| IBIS file stm32u575_585_ufbga132.ibs
[IBIS ver] 4.2
[File name] stm32u575_585_ufbga132.ibs
[File Rev] 1.0
[Date]   06-08-2021
[Source] Data Created at STMicroelectronics
[Notes]  File originated from ELDO simulations.
[Disclaimer]  This information is for modeling purpose only and is
   not guaranted. The information is subject to change without
   notice.
[Copyright] Copyright 2021 STMicroelectronics Inc.
|   Component stm32u575_585_ufbga132
[Component] stm32u575_585_ufbga132
[Manufacturer] STMicroelectronics
[Package]
| variable   typ   min   max
R_pkg   0   NA   NA
L_pkg   0   NA   NA
C_pkg   0   NA   NA
[Pin]   signal_name   model_name   R_pin   L_pin   C_pin   | Comment
A1 PE5 io8_100m_hslv_tamp_ft
A10 PC11 io8_100m_hslv_ft
A11 PA15 nc
A12 VDDUSB POWER
A2 PE3 io8_100m_hslv_tamp_ft
A3 PE1 io8_100m_hslv_ft
A4 PB9 io8_100m_i2c_ft
A5 PB6 io8_100m_i2c_ft
A6 PG12 io8_100m_hslv_ft
A7 PD6 io8_166m_hslv_ft
A8 PD5 io8_100m_hslv_ft
A9 PD2 io8_100m_ft
B1 VBAT POWER
B10 PC12 io8_166m_hslv_ft
B11 PC10 io8_100m_ft
B12 PA12 io8_usb_ft
B2 PE4 io8_100m_hslv_tamp_ft
B3 PE2 io8_100m_hslv_ft
B4 PG15 io8_100m_hslv_ft
B5 PH3-BOOT0 io8_100m_ft
B6 PB4 io8_100m_i2c_ft
B7 PG9 io8_100m_hslv_ft
B8 PD4 io8_100m_hslv_ft
B9 PD1 io8_100m_hslv_ft
C1 PC14-OSC32_IN io8_100m_ft
C10 PA13 io8_100m_ft
C11 PA14 io8_100m_ft
C12 PA11 io8_usb_ft
C2 PE6 io8_100m_hslv_tamp_ft
C3 PC13 io8_100m_ft_v33
C4 PE0 io8_100m_hslv_ft
C5 PB8 io8_100m_i2c_ft
C6 PB3 io8_100m_i2c_ft
C7 PG10 io8_100m_hslv_ft
C8 PD3 io8_166m_hslv_ft
C9 PD0 io8_100m_hslv_ft
D1 PC15-OSC32_OUT io8_100m_ft
D10 PA9 io8_100m_usb_vbus_ft
D11 PA10 io8_100m_usb_id
D12 PA8 io8_166m_hslv_ft
D2 PF0 io8_100m_hslv_ft
D3 PF3 io8_100m_hslv_ft
D4 VDD POWER
D5 PB7 io8_166m_hslv_i2c_ft
D6 PB5 io8_166m_hslv_ft
D7 PD7 io8_100m_hslv_ft
D8 VDDIO2 POWER
D9 VDD POWER
E1 PF2 io8_100m_hslv_ft
E10 PC7 io8_100m_ft
E11 PC9 io8_100m_ft
E12 PC8 io8_100m_ft
E2 PF1 io8_100m_hslv_ft
E3 PF4 io8_166m_hslv_ft
E4 VSS GND
E9 VSS GND
F1 PH0-OSC_IN io8_100m_ft
F10 PG7 io8_100m_hslv_ft
F11 PC6 io8_100m_ft
F12 PG8 io8_100m_i2c_ft
F2 PF5 io8_166m_hslv_ft
F3 PC2 io8_100m_hslv_ft
F4 PC3 io8_100m_hslv_ft
F6 VSS GND
F7 VDD POWER
F9 PG6 io8_100m_hslv_ft
G1 PH1-OSC_OUT io8_100m_ft
G10 PG2 io8_100m_hslv_ft
G11 PG3 io8_100m_hslv_ft
G12 PG5 io8_100m_hslv_ft
G2 NRST nc
G3 PC1 io8_166m_hslv_i2c_ft
G4 PA1 io8_100m_hslv_tamp_ft
G6 VDD POWER
G7 VSS GND
G9 PG4 io8_100m_hslv_ft
H1 VSSA GND
H10 PD14 io8_100m_hslv_ft
H11 PD13 io8_100m_hslv_ft
H12 PD15 io8_100m_hslv_ft
H2 PC0 io8_100m_hslv_ft
H3 OPAMP1_VINM nc
H4 VSS GND
H9 VSS GND
J1 VREF+ POWER
J10 PD9 io8_100m_hslv_ft
J11 PD11 io8_100m_hslv_ft
J12 PD12 io8_100m_hslv_ft
J2 PA0 io8_100m_hslv_tamp_ft
J3 PC5 io8_100m_tamp_ft
J4 VDD POWER
J5 PF14 io8_100m_hslv_ft
J6 PE8 io8_100m_hslv_ft
J7 PE10 io8_166m_hslv_ft
J8 PE12 io8_100m_hslv_ft
J9 VDD POWER
K1 VDDA POWER
K10 PB13 io8_100m_i2c_ft
K11 PB14 io8_100m_i2c_ft
K12 PB15 nc
K2 PA2 io8_100m_hslv_ft
K3 PA7 io8_100m_hslv_ft
K4 PB2 io8_100m_hslv_tamp_ft
K5 PF11 io8_166m_hslv_ft
K6 PG1 io8_100m_hslv_ft
K7 PE7 io8_100m_hslv_ft
K8 PE14 io8_100m_hslv_ft
K9 PB10 io8_166m_hslv_i2c_ft
L1 PA3 io8_166m_hslv_ft
L10 VCAP POWER
L11 PB12 io8_166m_hslv_ft
L12 PD8 io8_100m_hslv_ft
L2 PA6 io8_100m_hslv_ft
L3 PA4 io8_100m_hslv_ft
L4 PB1 io8_100m_hslv_ft
L5 PF12 io8_100m_hslv_ft
L6 PF15 io8_100m_hslv_ft
L7 PE11 io8_100m_hslv_ft
L8 PE15 io8_100m_hslv_ft
L9 PB11 io8_100m_hslv_ft
M1 PA5 io8_100m_ft
M10 PG13 io8_100m_hslv_ft
M11 PG11 io8_100m_hslv_ft
M12 PD10 io8_100m_hslv_ft
M2 OPAMP2_VINM nc
M3 PC4 io8_100m_hslv_ft
M4 PB0 io8_100m_hslv_ft
M5 PF13 io8_100m_hslv_ft
M6 PG0 io8_100m_hslv_ft
M7 PE9 io8_166m_hslv_ft
M8 PE13 io8_100m_hslv_ft
M9 PG14 io8_100m_hslv_ft
[Model Selector] io8_100m_ft
io8_100m_ft_hs_1v2  "IO8_FT 100MHz high speed @ 1.2V"
io8_100m_ft_hs_pu_1v2  "IO8_FT 100MHz high speed @ 1.2V pullup"
io8_100m_ft_hs_pd_1v2  "IO8_FT 100MHz high speed @ 1.2V pulldown"
io8_100m_ft_fs_1v2  "IO8_FT 100MHz fast speed @ 1.2V"
io8_100m_ft_fs_pu_1v2  "IO8_FT 100MHz fast speed @ 1.2V pullup"
io8_100m_ft_fs_pd_1v2  "IO8_FT 100MHz fast speed @ 1.2V pulldown"
io8_100m_ft_ms_1v2  "IO8_FT 100MHz med speed @ 1.2V"
io8_100m_ft_ms_pu_1v2  "IO8_FT 100MHz med speed @ 1.2V pullup"
io8_100m_ft_ms_pd_1v2  "IO8_FT 100MHz med speed @ 1.2V pulldown"
io8_100m_ft_ls_1v2  "IO8_FT 100MHz low speed @ 1.2V"
io8_100m_ft_ls_pu_1v2  "IO8_FT 100MHz low speed @ 1.2V pullup"
io8_100m_ft_ls_pd_1v2  "IO8_FT 100MHz low speed @ 1.2V pulldown"
io8_100m_ft_hs_1v8  "IO8_FT 100MHz high speed @ 1.8V"
io8_100m_ft_hs_pu_1v8  "IO8_FT 100MHz high speed @ 1.8V pullup"
io8_100m_ft_hs_pd_1v8  "IO8_FT 100MHz high speed @ 1.8V pulldown"
io8_100m_ft_fs_1v8  "IO8_FT 100MHz fast speed @ 1.8V"
io8_100m_ft_fs_pu_1v8  "IO8_FT 100MHz fast speed @ 1.8V pullup"
io8_100m_ft_fs_pd_1v8  "IO8_FT 100MHz fast speed @ 1.8V pulldown"
io8_100m_ft_ms_1v8  "IO8_FT 100MHz med speed @ 1.8V"
io8_100m_ft_ms_pu_1v8  "IO8_FT 100MHz med speed @ 1.8V pullup"
io8_100m_ft_ms_pd_1v8  "IO8_FT 100MHz med speed @ 1.8V pulldown"
io8_100m_ft_ls_1v8  "IO8_FT 100MHz low speed @ 1.8V"
io8_100m_ft_ls_pu_1v8  "IO8_FT 100MHz low speed @ 1.8V pullup"
io8_100m_ft_ls_pd_1v8  "IO8_FT 100MHz low speed @ 1.8V pulldown"
io8_100m_ft_hs_3v3  "IO8_FT 100MHz high speed @ 3.3V"
io8_100m_ft_hs_pu_3v3  "IO8_FT 100MHz high speed @ 3.3V pullup"
io8_100m_ft_hs_pd_3v3  "IO8_FT 100MHz high speed @ 3.3V pulldown"
io8_100m_ft_fs_3v3  "IO8_FT 100MHz fast speed @ 3.3V"
io8_100m_ft_fs_pu_3v3  "IO8_FT 100MHz fast speed @ 3.3V pullup"
io8_100m_ft_fs_pd_3v3  "IO8_FT 100MHz fast speed @ 3.3V pulldown"
io8_100m_ft_ms_3v3  "IO8_FT 100MHz med speed @ 3.3V"
io8_100m_ft_ms_pu_3v3  "IO8_FT 100MHz med speed @ 3.3V pullup"
io8_100m_ft_ms_pd_3v3  "IO8_FT 100MHz med speed @ 3.3V pulldown"
io8_100m_ft_ls_3v3  "IO8_FT 100MHz low speed @ 3.3V"
io8_100m_ft_ls_pu_3v3  "IO8_FT 100MHz low speed @ 3.3V pullup"
io8_100m_ft_ls_pd_3v3  "IO8_FT 100MHz low speed @ 3.3V pulldown"
[Model Selector] io8_100m_hslv_ft
io8_100m_ft_hs_1v2  "IO8_FT 100MHz high speed @ 1.2V"
io8_100m_ft_hs_pu_1v2  "IO8_FT 100MHz high speed @ 1.2V pullup"
io8_100m_ft_hs_pd_1v2  "IO8_FT 100MHz high speed @ 1.2V pulldown"
io8_100m_ft_fs_1v2  "IO8_FT 100MHz fast speed @ 1.2V"
io8_100m_ft_fs_pu_1v2  "IO8_FT 100MHz fast speed @ 1.2V pullup"
io8_100m_ft_fs_pd_1v2  "IO8_FT 100MHz fast speed @ 1.2V pulldown"
io8_100m_ft_ms_1v2  "IO8_FT 100MHz med speed @ 1.2V"
io8_100m_ft_ms_pu_1v2  "IO8_FT 100MHz med speed @ 1.2V pullup"
io8_100m_ft_ms_pd_1v2  "IO8_FT 100MHz med speed @ 1.2V pulldown"
io8_100m_ft_ls_1v2  "IO8_FT 100MHz low speed @ 1.2V"
io8_100m_ft_ls_pu_1v2  "IO8_FT 100MHz low speed @ 1.2V pullup"
io8_100m_ft_ls_pd_1v2  "IO8_FT 100MHz low speed @ 1.2V pulldown"
io8_100m_ft_hs_1v8  "IO8_FT 100MHz high speed @ 1.8V"
io8_100m_ft_hs_pu_1v8  "IO8_FT 100MHz high speed @ 1.8V pullup"
io8_100m_ft_hs_pd_1v8  "IO8_FT 100MHz high speed @ 1.8V pulldown"
io8_100m_ft_fs_1v8  "IO8_FT 100MHz fast speed @ 1.8V"
io8_100m_ft_fs_pu_1v8  "IO8_FT 100MHz fast speed @ 1.8V pullup"
io8_100m_ft_fs_pd_1v8  "IO8_FT 100MHz fast speed @ 1.8V pulldown"
io8_100m_ft_ms_1v8  "IO8_FT 100MHz med speed @ 1.8V"
io8_100m_ft_ms_pu_1v8  "IO8_FT 100MHz med speed @ 1.8V pullup"
io8_100m_ft_ms_pd_1v8  "IO8_FT 100MHz med speed @ 1.8V pulldown"
io8_100m_ft_ls_1v8  "IO8_FT 100MHz low speed @ 1.8V"
io8_100m_ft_ls_pu_1v8  "IO8_FT 100MHz low speed @ 1.8V pullup"
io8_100m_ft_ls_pd_1v8  "IO8_FT 100MHz low speed @ 1.8V pulldown"
io8_100m_ft_hs_3v3  "IO8_FT 100MHz high speed @ 3.3V"
io8_100m_ft_hs_pu_3v3  "IO8_FT 100MHz high speed @ 3.3V pullup"
io8_100m_ft_hs_pd_3v3  "IO8_FT 100MHz high speed @ 3.3V pulldown"
io8_100m_ft_fs_3v3  "IO8_FT 100MHz fast speed @ 3.3V"
io8_100m_ft_fs_pu_3v3  "IO8_FT 100MHz fast speed @ 3.3V pullup"
io8_100m_ft_fs_pd_3v3  "IO8_FT 100MHz fast speed @ 3.3V pulldown"
io8_100m_ft_ms_3v3  "IO8_FT 100MHz med speed @ 3.3V"
io8_100m_ft_ms_pu_3v3  "IO8_FT 100MHz med speed @ 3.3V pullup"
io8_100m_ft_ms_pd_3v3  "IO8_FT 100MHz med speed @ 3.3V pulldown"
io8_100m_ft_ls_3v3  "IO8_FT 100MHz low speed @ 3.3V"
io8_100m_ft_ls_pu_3v3  "IO8_FT 100MHz low speed @ 3.3V pullup"
io8_100m_ft_ls_pd_3v3  "IO8_FT 100MHz low speed @ 3.3V pulldown"
io8_100m_hslv_ft_hs_1v2  "IO8_FT 100MHz HSLV high speed @ 1.2V"
io8_100m_hslv_ft_hs_pu_1v2  "IO8_FT 100MHz HSLV high speed @ 1.2V pullup"
io8_100m_hslv_ft_hs_pd_1v2  "IO8_FT 100MHz HSLV high speed @ 1.2V pulldown"
io8_100m_hslv_ft_fs_1v2  "IO8_FT 100MHz HSLV fast speed @ 1.2V"
io8_100m_hslv_ft_fs_pu_1v2  "IO8_FT 100MHz HSLV fast speed @ 1.2V pullup"
io8_100m_hslv_ft_fs_pd_1v2  "IO8_FT 100MHz HSLV fast speed @ 1.2V pulldown"
io8_100m_hslv_ft_ms_1v2  "IO8_FT 100MHz HSLV med speed @ 1.2V"
io8_100m_hslv_ft_ms_pu_1v2  "IO8_FT 100MHz HSLV med speed @ 1.2V pullup"
io8_100m_hslv_ft_ms_pd_1v2  "IO8_FT 100MHz HSLV med speed @ 1.2V pulldown"
io8_100m_hslv_ft_ls_1v2  "IO8_FT 100MHz HSLV low speed @ 1.2V"
io8_100m_hslv_ft_ls_pu_1v2  "IO8_FT 100MHz HSLV low speed @ 1.2V pullup"
io8_100m_hslv_ft_ls_pd_1v2  "IO8_FT 100MHz HSLV low speed @ 1.2V pulldown"
io8_100m_hslv_ft_hs_1v8  "IO8_FT 100MHz HSLV high speed @ 1.8V"
io8_100m_hslv_ft_hs_pu_1v8  "IO8_FT 100MHz HSLV high speed @ 1.8V pullup"
io8_100m_hslv_ft_hs_pd_1v8  "IO8_FT 100MHz HSLV high speed @ 1.8V pulldown"
io8_100m_hslv_ft_fs_1v8  "IO8_FT 100MHz HSLV fast speed @ 1.8V"
io8_100m_hslv_ft_fs_pu_1v8  "IO8_FT 100MHz HSLV fast speed @ 1.8V pullup"
io8_100m_hslv_ft_fs_pd_1v8  "IO8_FT 100MHz HSLV fast speed @ 1.8V pulldown"
io8_100m_hslv_ft_ms_1v8  "IO8_FT 100MHz HSLV med speed @ 1.8V"
io8_100m_hslv_ft_ms_pu_1v8  "IO8_FT 100MHz HSLV med speed @ 1.8V pullup"
io8_100m_hslv_ft_ms_pd_1v8  "IO8_FT 100MHz HSLV med speed @ 1.8V pulldown"
io8_100m_hslv_ft_ls_1v8  "IO8_FT 100MHz HSLV low speed @ 1.8V"
io8_100m_hslv_ft_ls_pu_1v8  "IO8_FT 100MHz HSLV low speed @ 1.8V pullup"
io8_100m_hslv_ft_ls_pd_1v8  "IO8_FT 100MHz HSLV low speed @ 1.8V pulldown"
io8_100m_hslv_ft_hs_2v5  "IO8_FT 100MHz HSLV high speed @ 2.5V"
io8_100m_hslv_ft_hs_pu_2v5  "IO8_FT 100MHz HSLV high speed @ 2.5V pullup"
io8_100m_hslv_ft_hs_pd_2v5  "IO8_FT 100MHz HSLV high speed @ 2.5V pulldown"
io8_100m_hslv_ft_fs_2v5  "IO8_FT 100MHz HSLV fast speed @ 2.5V"
io8_100m_hslv_ft_fs_pu_2v5  "IO8_FT 100MHz HSLV fast speed @ 2.5V pullup"
io8_100m_hslv_ft_fs_pd_2v5  "IO8_FT 100MHz HSLV fast speed @ 2.5V pulldown"
io8_100m_hslv_ft_ms_2v5  "IO8_FT 100MHz HSLV med speed @ 2.5V"
io8_100m_hslv_ft_ms_pu_2v5  "IO8_FT 100MHz HSLV med speed @ 2.5V pullup"
io8_100m_hslv_ft_ms_pd_2v5  "IO8_FT 100MHz HSLV med speed @ 2.5V pulldown"
io8_100m_hslv_ft_ls_2v5  "IO8_FT 100MHz HSLV low speed @ 2.5V"
io8_100m_hslv_ft_ls_pu_2v5  "IO8_FT 100MHz HSLV low speed @ 2.5V pullup"
io8_100m_hslv_ft_ls_pd_2v5  "IO8_FT 100MHz HSLV low speed @ 2.5V pulldown"
[Model Selector] io8_166m_hslv_ft
io8_166m_ft_hs_1v2  "IO8_FT 166MHz high speed @ 1.2V"
io8_166m_ft_hs_pu_1v2  "IO8_FT 166MHz high speed @ 1.2V pullup"
io8_166m_ft_hs_pd_1v2  "IO8_FT 166MHz high speed @ 1.2V pulldown"
io8_166m_ft_fs_1v2  "IO8_FT 166MHz fast speed @ 1.2V"
io8_166m_ft_fs_pu_1v2  "IO8_FT 166MHz fast speed @ 1.2V pullup"
io8_166m_ft_fs_pd_1v2  "IO8_FT 166MHz fast speed @ 1.2V pulldown"
io8_166m_ft_ms_1v2  "IO8_FT 166MHz med speed @ 1.2V"
io8_166m_ft_ms_pu_1v2  "IO8_FT 166MHz med speed @ 1.2V pullup"
io8_166m_ft_ms_pd_1v2  "IO8_FT 166MHz med speed @ 1.2V pulldown"
io8_166m_ft_ls_1v2  "IO8_FT 166MHz low speed @ 1.2V"
io8_166m_ft_ls_pu_1v2  "IO8_FT 166MHz low speed @ 1.2V pullup"
io8_166m_ft_ls_pd_1v2  "IO8_FT 166MHz low speed @ 1.2V pulldown"
io8_166m_ft_hs_1v8  "IO8_FT 166MHz high speed @ 1.8V"
io8_166m_ft_hs_pu_1v8  "IO8_FT 166MHz high speed @ 1.8V pullup"
io8_166m_ft_hs_pd_1v8  "IO8_FT 166MHz high speed @ 1.8V pulldown"
io8_166m_ft_fs_1v8  "IO8_FT 166MHz fast speed @ 1.8V"
io8_166m_ft_fs_pu_1v8  "IO8_FT 166MHz fast speed @ 1.8V pullup"
io8_166m_ft_fs_pd_1v8  "IO8_FT 166MHz fast speed @ 1.8V pulldown"
io8_166m_ft_ms_1v8  "IO8_FT 166MHz med speed @ 1.8V"
io8_166m_ft_ms_pu_1v8  "IO8_FT 166MHz med speed @ 1.8V pullup"
io8_166m_ft_ms_pd_1v8  "IO8_FT 166MHz med speed @ 1.8V pulldown"
io8_166m_ft_ls_1v8  "IO8_FT 166MHz low speed @ 1.8V"
io8_166m_ft_ls_pu_1v8  "IO8_FT 166MHz low speed @ 1.8V pullup"
io8_166m_ft_ls_pd_1v8  "IO8_FT 166MHz low speed @ 1.8V pulldown"
io8_166m_ft_hs_3v3  "IO8_FT 166MHz high speed @ 3.3V"
io8_166m_ft_hs_pu_3v3  "IO8_FT 166MHz high speed @ 3.3V pullup"
io8_166m_ft_hs_pd_3v3  "IO8_FT 166MHz high speed @ 3.3V pulldown"
io8_166m_ft_fs_3v3  "IO8_FT 166MHz fast speed @ 3.3V"
io8_166m_ft_fs_pu_3v3  "IO8_FT 166MHz fast speed @ 3.3V pullup"
io8_166m_ft_fs_pd_3v3  "IO8_FT 166MHz fast speed @ 3.3V pulldown"
io8_166m_ft_ms_3v3  "IO8_FT 166MHz med speed @ 3.3V"
io8_166m_ft_ms_pu_3v3  "IO8_FT 166MHz med speed @ 3.3V pullup"
io8_166m_ft_ms_pd_3v3  "IO8_FT 166MHz med speed @ 3.3V pulldown"
io8_166m_ft_ls_3v3  "IO8_FT 166MHz low speed @ 3.3V"
io8_166m_ft_ls_pu_3v3  "IO8_FT 166MHz low speed @ 3.3V pullup"
io8_166m_ft_ls_pd_3v3  "IO8_FT 166MHz low speed @ 3.3V pulldown"
io8_166m_hslv_ft_hs_1v2  "IO8_FT 166MHz HSLV high speed @ 1.2V"
io8_166m_hslv_ft_hs_pu_1v2  "IO8_FT 166MHz HSLV high speed @ 1.2V pullup"
io8_166m_hslv_ft_hs_pd_1v2  "IO8_FT 166MHz HSLV high speed @ 1.2V pulldown"
io8_166m_hslv_ft_fs_1v2  "IO8_FT 166MHz HSLV fast speed @ 1.2V"
io8_166m_hslv_ft_fs_pu_1v2  "IO8_FT 166MHz HSLV fast speed @ 1.2V pullup"
io8_166m_hslv_ft_fs_pd_1v2  "IO8_FT 166MHz HSLV fast speed @ 1.2V pulldown"
io8_166m_hslv_ft_ms_1v2  "IO8_FT 166MHz HSLV med speed @ 1.2V"
io8_166m_hslv_ft_ms_pu_1v2  "IO8_FT 166MHz HSLV med speed @ 1.2V pullup"
io8_166m_hslv_ft_ms_pd_1v2  "IO8_FT 166MHz HSLV med speed @ 1.2V pulldown"
io8_166m_hslv_ft_ls_1v2  "IO8_FT 166MHz HSLV low speed @ 1.2V"
io8_166m_hslv_ft_ls_pu_1v2  "IO8_FT 166MHz HSLV low speed @ 1.2V pullup"
io8_166m_hslv_ft_ls_pd_1v2  "IO8_FT 166MHz HSLV low speed @ 1.2V pulldown"
io8_166m_hslv_ft_hs_1v8  "IO8_FT 166MHz HSLV high speed @ 1.8V"
io8_166m_hslv_ft_hs_pu_1v8  "IO8_FT 166MHz HSLV high speed @ 1.8V pullup"
io8_166m_hslv_ft_hs_pd_1v8  "IO8_FT 166MHz HSLV high speed @ 1.8V pulldown"
io8_166m_hslv_ft_fs_1v8  "IO8_FT 166MHz HSLV fast speed @ 1.8V"
io8_166m_hslv_ft_fs_pu_1v8  "IO8_FT 166MHz HSLV fast speed @ 1.8V pullup"
io8_166m_hslv_ft_fs_pd_1v8  "IO8_FT 166MHz HSLV fast speed @ 1.8V pulldown"
io8_166m_hslv_ft_ms_1v8  "IO8_FT 166MHz HSLV med speed @ 1.8V"
io8_166m_hslv_ft_ms_pu_1v8  "IO8_FT 166MHz HSLV med speed @ 1.8V pullup"
io8_166m_hslv_ft_ms_pd_1v8  "IO8_FT 166MHz HSLV med speed @ 1.8V pulldown"
io8_166m_hslv_ft_ls_1v8  "IO8_FT 166MHz HSLV low speed @ 1.8V"
io8_166m_hslv_ft_ls_pu_1v8  "IO8_FT 166MHz HSLV low speed @ 1.8V pullup"
io8_166m_hslv_ft_ls_pd_1v8  "IO8_FT 166MHz HSLV low speed @ 1.8V pulldown"
io8_166m_hslv_ft_hs_2v5  "IO8_FT 166MHz HSLV high speed @ 2.5V"
io8_166m_hslv_ft_hs_pu_2v5  "IO8_FT 166MHz HSLV high speed @ 2.5V pullup"
io8_166m_hslv_ft_hs_pd_2v5  "IO8_FT 166MHz HSLV high speed @ 2.5V pulldown"
io8_166m_hslv_ft_fs_2v5  "IO8_FT 166MHz HSLV fast speed @ 2.5V"
io8_166m_hslv_ft_fs_pu_2v5  "IO8_FT 166MHz HSLV fast speed @ 2.5V pullup"
io8_166m_hslv_ft_fs_pd_2v5  "IO8_FT 166MHz HSLV fast speed @ 2.5V pulldown"
io8_166m_hslv_ft_ms_2v5  "IO8_FT 166MHz HSLV med speed @ 2.5V"
io8_166m_hslv_ft_ms_pu_2v5  "IO8_FT 166MHz HSLV med speed @ 2.5V pullup"
io8_166m_hslv_ft_ms_pd_2v5  "IO8_FT 166MHz HSLV med speed @ 2.5V pulldown"
io8_166m_hslv_ft_ls_2v5  "IO8_FT 166MHz HSLV low speed @ 2.5V"
io8_166m_hslv_ft_ls_pu_2v5  "IO8_FT 166MHz HSLV low speed @ 2.5V pullup"
io8_166m_hslv_ft_ls_pd_2v5  "IO8_FT 166MHz HSLV low speed @ 2.5V pulldown"
[Model Selector] io8_100m_ft_v33
io8_ft_v33_hs_1v2  "IO8_FT_V33 high speed @ 1.2V"
io8_ft_v33_hs_pu_1v2  "IO8_FT_V33 high speed @ 1.2V pullup"
io8_ft_v33_hs_pd_1v2  "IO8_FT_V33 high speed @ 1.2V pulldown"
io8_ft_v33_fs_1v2  "IO8_FT_V33 fast speed @ 1.2V"
io8_ft_v33_fs_pu_1v2  "IO8_FT_V33 fast speed @ 1.2V pullup"
io8_ft_v33_fs_pd_1v2  "IO8_FT_V33 fast speed @ 1.2V pulldown"
io8_ft_v33_ms_1v2  "IO8_FT_V33 med speed @ 1.2V"
io8_ft_v33_ms_pu_1v2  "IO8_FT_V33 med speed @ 1.2V pullup"
io8_ft_v33_ms_pd_1v2  "IO8_FT_V33 med speed @ 1.2V pulldown"
io8_ft_v33_ls_1v2  "IO8_FT_V33 low speed @ 1.2V"
io8_ft_v33_ls_pu_1v2  "IO8_FT_V33 low speed @ 1.2V pullup"
io8_ft_v33_ls_pd_1v2  "IO8_FT_V33 low speed @ 1.2V pulldown"
io8_ft_v33_hs_1v8  "IO8_FT_V33 high speed @ 1.8V"
io8_ft_v33_hs_pu_1v8  "IO8_FT_V33 high speed @ 1.8V pullup"
io8_ft_v33_hs_pd_1v8  "IO8_FT_V33 high speed @ 1.8V pulldown"
io8_ft_v33_fs_1v8  "IO8_FT_V33 fast speed @ 1.8V"
io8_ft_v33_fs_pu_1v8  "IO8_FT_V33 fast speed @ 1.8V pullup"
io8_ft_v33_fs_pd_1v8  "IO8_FT_V33 fast speed @ 1.8V pulldown"
io8_ft_v33_ms_1v8  "IO8_FT_V33 med speed @ 1.8V"
io8_ft_v33_ms_pu_1v8  "IO8_FT_V33 med speed @ 1.8V pullup"
io8_ft_v33_ms_pd_1v8  "IO8_FT_V33 med speed @ 1.8V pulldown"
io8_ft_v33_ls_1v8  "IO8_FT_V33 low speed @ 1.8V"
io8_ft_v33_ls_pu_1v8  "IO8_FT_V33 low speed @ 1.8V pullup"
io8_ft_v33_ls_pd_1v8  "IO8_FT_V33 low speed @ 1.8V pulldown"
io8_ft_v33_hs_3v3  "IO8_FT_V33 high speed @ 3.3V"
io8_ft_v33_hs_pu_3v3  "IO8_FT_V33 high speed @ 3.3V pullup"
io8_ft_v33_hs_pd_3v3  "IO8_FT_V33 high speed @ 3.3V pulldown"
io8_ft_v33_fs_3v3  "IO8_FT_V33 fast speed @ 3.3V"
io8_ft_v33_fs_pu_3v3  "IO8_FT_V33 fast speed @ 3.3V pullup"
io8_ft_v33_fs_pd_3v3  "IO8_FT_V33 fast speed @ 3.3V pulldown"
io8_ft_v33_ms_3v3  "IO8_FT_V33 med speed @ 3.3V"
io8_ft_v33_ms_pu_3v3  "IO8_FT_V33 med speed @ 3.3V pullup"
io8_ft_v33_ms_pd_3v3  "IO8_FT_V33 med speed @ 3.3V pulldown"
io8_ft_v33_ls_3v3  "IO8_FT_V33 low speed @ 3.3V"
io8_ft_v33_ls_pu_3v3  "IO8_FT_V33 low speed @ 3.3V pullup"
io8_ft_v33_ls_pd_3v3  "IO8_FT_V33 low speed @ 3.3V pulldown"
[Model Selector] io8_100m_tamp_ft
io8_100m_ft_hs_1v2  "IO8_FT 100MHz high speed @ 1.2V"
io8_100m_ft_hs_pu_1v2  "IO8_FT 100MHz high speed @ 1.2V pullup"
io8_100m_ft_hs_pd_1v2  "IO8_FT 100MHz high speed @ 1.2V pulldown"
io8_100m_ft_fs_1v2  "IO8_FT 100MHz fast speed @ 1.2V"
io8_100m_ft_fs_pu_1v2  "IO8_FT 100MHz fast speed @ 1.2V pullup"
io8_100m_ft_fs_pd_1v2  "IO8_FT 100MHz fast speed @ 1.2V pulldown"
io8_100m_ft_ms_1v2  "IO8_FT 100MHz med speed @ 1.2V"
io8_100m_ft_ms_pu_1v2  "IO8_FT 100MHz med speed @ 1.2V pullup"
io8_100m_ft_ms_pd_1v2  "IO8_FT 100MHz med speed @ 1.2V pulldown"
io8_100m_ft_ls_1v2  "IO8_FT 100MHz low speed @ 1.2V"
io8_100m_ft_ls_pu_1v2  "IO8_FT 100MHz low speed @ 1.2V pullup"
io8_100m_ft_ls_pd_1v2  "IO8_FT 100MHz low speed @ 1.2V pulldown"
io8_100m_ft_hs_1v8  "IO8_FT 100MHz high speed @ 1.8V"
io8_100m_ft_hs_pu_1v8  "IO8_FT 100MHz high speed @ 1.8V pullup"
io8_100m_ft_hs_pd_1v8  "IO8_FT 100MHz high speed @ 1.8V pulldown"
io8_100m_ft_fs_1v8  "IO8_FT 100MHz fast speed @ 1.8V"
io8_100m_ft_fs_pu_1v8  "IO8_FT 100MHz fast speed @ 1.8V pullup"
io8_100m_ft_fs_pd_1v8  "IO8_FT 100MHz fast speed @ 1.8V pulldown"
io8_100m_ft_ms_1v8  "IO8_FT 100MHz med speed @ 1.8V"
io8_100m_ft_ms_pu_1v8  "IO8_FT 100MHz med speed @ 1.8V pullup"
io8_100m_ft_ms_pd_1v8  "IO8_FT 100MHz med speed @ 1.8V pulldown"
io8_100m_ft_ls_1v8  "IO8_FT 100MHz low speed @ 1.8V"
io8_100m_ft_ls_pu_1v8  "IO8_FT 100MHz low speed @ 1.8V pullup"
io8_100m_ft_ls_pd_1v8  "IO8_FT 100MHz low speed @ 1.8V pulldown"
io8_100m_ft_hs_3v3  "IO8_FT 100MHz high speed @ 3.3V"
io8_100m_ft_hs_pu_3v3  "IO8_FT 100MHz high speed @ 3.3V pullup"
io8_100m_ft_hs_pd_3v3  "IO8_FT 100MHz high speed @ 3.3V pulldown"
io8_100m_ft_fs_3v3  "IO8_FT 100MHz fast speed @ 3.3V"
io8_100m_ft_fs_pu_3v3  "IO8_FT 100MHz fast speed @ 3.3V pullup"
io8_100m_ft_fs_pd_3v3  "IO8_FT 100MHz fast speed @ 3.3V pulldown"
io8_100m_ft_ms_3v3  "IO8_FT 100MHz med speed @ 3.3V"
io8_100m_ft_ms_pu_3v3  "IO8_FT 100MHz med speed @ 3.3V pullup"
io8_100m_ft_ms_pd_3v3  "IO8_FT 100MHz med speed @ 3.3V pulldown"
io8_100m_ft_ls_3v3  "IO8_FT 100MHz low speed @ 3.3V"
io8_100m_ft_ls_pu_3v3  "IO8_FT 100MHz low speed @ 3.3V pullup"
io8_100m_ft_ls_pd_3v3  "IO8_FT 100MHz low speed @ 3.3V pulldown"
io8_ft_v33_hs_1v2  "IO8_FT_V33 high speed @ 1.2V"
io8_ft_v33_hs_pu_1v2  "IO8_FT_V33 high speed @ 1.2V pullup"
io8_ft_v33_hs_pd_1v2  "IO8_FT_V33 high speed @ 1.2V pulldown"
io8_ft_v33_fs_1v2  "IO8_FT_V33 fast speed @ 1.2V"
io8_ft_v33_fs_pu_1v2  "IO8_FT_V33 fast speed @ 1.2V pullup"
io8_ft_v33_fs_pd_1v2  "IO8_FT_V33 fast speed @ 1.2V pulldown"
io8_ft_v33_ms_1v2  "IO8_FT_V33 med speed @ 1.2V"
io8_ft_v33_ms_pu_1v2  "IO8_FT_V33 med speed @ 1.2V pullup"
io8_ft_v33_ms_pd_1v2  "IO8_FT_V33 med speed @ 1.2V pulldown"
io8_ft_v33_ls_1v2  "IO8_FT_V33 low speed @ 1.2V"
io8_ft_v33_ls_pu_1v2  "IO8_FT_V33 low speed @ 1.2V pullup"
io8_ft_v33_ls_pd_1v2  "IO8_FT_V33 low speed @ 1.2V pulldown"
io8_ft_v33_hs_1v8  "IO8_FT_V33 high speed @ 1.8V"
io8_ft_v33_hs_pu_1v8  "IO8_FT_V33 high speed @ 1.8V pullup"
io8_ft_v33_hs_pd_1v8  "IO8_FT_V33 high speed @ 1.8V pulldown"
io8_ft_v33_fs_1v8  "IO8_FT_V33 fast speed @ 1.8V"
io8_ft_v33_fs_pu_1v8  "IO8_FT_V33 fast speed @ 1.8V pullup"
io8_ft_v33_fs_pd_1v8  "IO8_FT_V33 fast speed @ 1.8V pulldown"
io8_ft_v33_ms_1v8  "IO8_FT_V33 med speed @ 1.8V"
io8_ft_v33_ms_pu_1v8  "IO8_FT_V33 med speed @ 1.8V pullup"
io8_ft_v33_ms_pd_1v8  "IO8_FT_V33 med speed @ 1.8V pulldown"
io8_ft_v33_ls_1v8  "IO8_FT_V33 low speed @ 1.8V"
io8_ft_v33_ls_pu_1v8  "IO8_FT_V33 low speed @ 1.8V pullup"
io8_ft_v33_ls_pd_1v8  "IO8_FT_V33 low speed @ 1.8V pulldown"
io8_ft_v33_hs_3v3  "IO8_FT_V33 high speed @ 3.3V"
io8_ft_v33_hs_pu_3v3  "IO8_FT_V33 high speed @ 3.3V pullup"
io8_ft_v33_hs_pd_3v3  "IO8_FT_V33 high speed @ 3.3V pulldown"
io8_ft_v33_fs_3v3  "IO8_FT_V33 fast speed @ 3.3V"
io8_ft_v33_fs_pu_3v3  "IO8_FT_V33 fast speed @ 3.3V pullup"
io8_ft_v33_fs_pd_3v3  "IO8_FT_V33 fast speed @ 3.3V pulldown"
io8_ft_v33_ms_3v3  "IO8_FT_V33 med speed @ 3.3V"
io8_ft_v33_ms_pu_3v3  "IO8_FT_V33 med speed @ 3.3V pullup"
io8_ft_v33_ms_pd_3v3  "IO8_FT_V33 med speed @ 3.3V pulldown"
io8_ft_v33_ls_3v3  "IO8_FT_V33 low speed @ 3.3V"
io8_ft_v33_ls_pu_3v3  "IO8_FT_V33 low speed @ 3.3V pullup"
io8_ft_v33_ls_pd_3v3  "IO8_FT_V33 low speed @ 3.3V pulldown"
[Model Selector] io8_100m_hslv_tamp_ft
io8_100m_ft_hs_1v2  "IO8_FT 100MHz high speed @ 1.2V"
io8_100m_ft_hs_pu_1v2  "IO8_FT 100MHz high speed @ 1.2V pullup"
io8_100m_ft_hs_pd_1v2  "IO8_FT 100MHz high speed @ 1.2V pulldown"
io8_100m_ft_fs_1v2  "IO8_FT 100MHz fast speed @ 1.2V"
io8_100m_ft_fs_pu_1v2  "IO8_FT 100MHz fast speed @ 1.2V pullup"
io8_100m_ft_fs_pd_1v2  "IO8_FT 100MHz fast speed @ 1.2V pulldown"
io8_100m_ft_ms_1v2  "IO8_FT 100MHz med speed @ 1.2V"
io8_100m_ft_ms_pu_1v2  "IO8_FT 100MHz med speed @ 1.2V pullup"
io8_100m_ft_ms_pd_1v2  "IO8_FT 100MHz med speed @ 1.2V pulldown"
io8_100m_ft_ls_1v2  "IO8_FT 100MHz low speed @ 1.2V"
io8_100m_ft_ls_pu_1v2  "IO8_FT 100MHz low speed @ 1.2V pullup"
io8_100m_ft_ls_pd_1v2  "IO8_FT 100MHz low speed @ 1.2V pulldown"
io8_100m_ft_hs_1v8  "IO8_FT 100MHz high speed @ 1.8V"
io8_100m_ft_hs_pu_1v8  "IO8_FT 100MHz high speed @ 1.8V pullup"
io8_100m_ft_hs_pd_1v8  "IO8_FT 100MHz high speed @ 1.8V pulldown"
io8_100m_ft_fs_1v8  "IO8_FT 100MHz fast speed @ 1.8V"
io8_100m_ft_fs_pu_1v8  "IO8_FT 100MHz fast speed @ 1.8V pullup"
io8_100m_ft_fs_pd_1v8  "IO8_FT 100MHz fast speed @ 1.8V pulldown"
io8_100m_ft_ms_1v8  "IO8_FT 100MHz med speed @ 1.8V"
io8_100m_ft_ms_pu_1v8  "IO8_FT 100MHz med speed @ 1.8V pullup"
io8_100m_ft_ms_pd_1v8  "IO8_FT 100MHz med speed @ 1.8V pulldown"
io8_100m_ft_ls_1v8  "IO8_FT 100MHz low speed @ 1.8V"
io8_100m_ft_ls_pu_1v8  "IO8_FT 100MHz low speed @ 1.8V pullup"
io8_100m_ft_ls_pd_1v8  "IO8_FT 100MHz low speed @ 1.8V pulldown"
io8_100m_ft_hs_3v3  "IO8_FT 100MHz high speed @ 3.3V"
io8_100m_ft_hs_pu_3v3  "IO8_FT 100MHz high speed @ 3.3V pullup"
io8_100m_ft_hs_pd_3v3  "IO8_FT 100MHz high speed @ 3.3V pulldown"
io8_100m_ft_fs_3v3  "IO8_FT 100MHz fast speed @ 3.3V"
io8_100m_ft_fs_pu_3v3  "IO8_FT 100MHz fast speed @ 3.3V pullup"
io8_100m_ft_fs_pd_3v3  "IO8_FT 100MHz fast speed @ 3.3V pulldown"
io8_100m_ft_ms_3v3  "IO8_FT 100MHz med speed @ 3.3V"
io8_100m_ft_ms_pu_3v3  "IO8_FT 100MHz med speed @ 3.3V pullup"
io8_100m_ft_ms_pd_3v3  "IO8_FT 100MHz med speed @ 3.3V pulldown"
io8_100m_ft_ls_3v3  "IO8_FT 100MHz low speed @ 3.3V"
io8_100m_ft_ls_pu_3v3  "IO8_FT 100MHz low speed @ 3.3V pullup"
io8_100m_ft_ls_pd_3v3  "IO8_FT 100MHz low speed @ 3.3V pulldown"
io8_100m_hslv_ft_hs_1v2  "IO8_FT 100MHz HSLV high speed @ 1.2V"
io8_100m_hslv_ft_hs_pu_1v2  "IO8_FT 100MHz HSLV high speed @ 1.2V pullup"
io8_100m_hslv_ft_hs_pd_1v2  "IO8_FT 100MHz HSLV high speed @ 1.2V pulldown"
io8_100m_hslv_ft_fs_1v2  "IO8_FT 100MHz HSLV fast speed @ 1.2V"
io8_100m_hslv_ft_fs_pu_1v2  "IO8_FT 100MHz HSLV fast speed @ 1.2V pullup"
io8_100m_hslv_ft_fs_pd_1v2  "IO8_FT 100MHz HSLV fast speed @ 1.2V pulldown"
io8_100m_hslv_ft_ms_1v2  "IO8_FT 100MHz HSLV med speed @ 1.2V"
io8_100m_hslv_ft_ms_pu_1v2  "IO8_FT 100MHz HSLV med speed @ 1.2V pullup"
io8_100m_hslv_ft_ms_pd_1v2  "IO8_FT 100MHz HSLV med speed @ 1.2V pulldown"
io8_100m_hslv_ft_ls_1v2  "IO8_FT 100MHz HSLV low speed @ 1.2V"
io8_100m_hslv_ft_ls_pu_1v2  "IO8_FT 100MHz HSLV low speed @ 1.2V pullup"
io8_100m_hslv_ft_ls_pd_1v2  "IO8_FT 100MHz HSLV low speed @ 1.2V pulldown"
io8_100m_hslv_ft_hs_1v8  "IO8_FT 100MHz HSLV high speed @ 1.8V"
io8_100m_hslv_ft_hs_pu_1v8  "IO8_FT 100MHz HSLV high speed @ 1.8V pullup"
io8_100m_hslv_ft_hs_pd_1v8  "IO8_FT 100MHz HSLV high speed @ 1.8V pulldown"
io8_100m_hslv_ft_fs_1v8  "IO8_FT 100MHz HSLV fast speed @ 1.8V"
io8_100m_hslv_ft_fs_pu_1v8  "IO8_FT 100MHz HSLV fast speed @ 1.8V pullup"
io8_100m_hslv_ft_fs_pd_1v8  "IO8_FT 100MHz HSLV fast speed @ 1.8V pulldown"
io8_100m_hslv_ft_ms_1v8  "IO8_FT 100MHz HSLV med speed @ 1.8V"
io8_100m_hslv_ft_ms_pu_1v8  "IO8_FT 100MHz HSLV med speed @ 1.8V pullup"
io8_100m_hslv_ft_ms_pd_1v8  "IO8_FT 100MHz HSLV med speed @ 1.8V pulldown"
io8_100m_hslv_ft_ls_1v8  "IO8_FT 100MHz HSLV low speed @ 1.8V"
io8_100m_hslv_ft_ls_pu_1v8  "IO8_FT 100MHz HSLV low speed @ 1.8V pullup"
io8_100m_hslv_ft_ls_pd_1v8  "IO8_FT 100MHz HSLV low speed @ 1.8V pulldown"
io8_100m_hslv_ft_hs_2v5  "IO8_FT 100MHz HSLV high speed @ 2.5V"
io8_100m_hslv_ft_hs_pu_2v5  "IO8_FT 100MHz HSLV high speed @ 2.5V pullup"
io8_100m_hslv_ft_hs_pd_2v5  "IO8_FT 100MHz HSLV high speed @ 2.5V pulldown"
io8_100m_hslv_ft_fs_2v5  "IO8_FT 100MHz HSLV fast speed @ 2.5V"
io8_100m_hslv_ft_fs_pu_2v5  "IO8_FT 100MHz HSLV fast speed @ 2.5V pullup"
io8_100m_hslv_ft_fs_pd_2v5  "IO8_FT 100MHz HSLV fast speed @ 2.5V pulldown"
io8_100m_hslv_ft_ms_2v5  "IO8_FT 100MHz HSLV med speed @ 2.5V"
io8_100m_hslv_ft_ms_pu_2v5  "IO8_FT 100MHz HSLV med speed @ 2.5V pullup"
io8_100m_hslv_ft_ms_pd_2v5  "IO8_FT 100MHz HSLV med speed @ 2.5V pulldown"
io8_100m_hslv_ft_ls_2v5  "IO8_FT 100MHz HSLV low speed @ 2.5V"
io8_100m_hslv_ft_ls_pu_2v5  "IO8_FT 100MHz HSLV low speed @ 2.5V pullup"
io8_100m_hslv_ft_ls_pd_2v5  "IO8_FT 100MHz HSLV low speed @ 2.5V pulldown"
io8_ft_v33_hs_1v2  "IO8_FT_V33 high speed @ 1.2V"
io8_ft_v33_hs_pu_1v2  "IO8_FT_V33 high speed @ 1.2V pullup"
io8_ft_v33_hs_pd_1v2  "IO8_FT_V33 high speed @ 1.2V pulldown"
io8_ft_v33_fs_1v2  "IO8_FT_V33 fast speed @ 1.2V"
io8_ft_v33_fs_pu_1v2  "IO8_FT_V33 fast speed @ 1.2V pullup"
io8_ft_v33_fs_pd_1v2  "IO8_FT_V33 fast speed @ 1.2V pulldown"
io8_ft_v33_ms_1v2  "IO8_FT_V33 med speed @ 1.2V"
io8_ft_v33_ms_pu_1v2  "IO8_FT_V33 med speed @ 1.2V pullup"
io8_ft_v33_ms_pd_1v2  "IO8_FT_V33 med speed @ 1.2V pulldown"
io8_ft_v33_ls_1v2  "IO8_FT_V33 low speed @ 1.2V"
io8_ft_v33_ls_pu_1v2  "IO8_FT_V33 low speed @ 1.2V pullup"
io8_ft_v33_ls_pd_1v2  "IO8_FT_V33 low speed @ 1.2V pulldown"
io8_ft_v33_hs_1v8  "IO8_FT_V33 high speed @ 1.8V"
io8_ft_v33_hs_pu_1v8  "IO8_FT_V33 high speed @ 1.8V pullup"
io8_ft_v33_hs_pd_1v8  "IO8_FT_V33 high speed @ 1.8V pulldown"
io8_ft_v33_fs_1v8  "IO8_FT_V33 fast speed @ 1.8V"
io8_ft_v33_fs_pu_1v8  "IO8_FT_V33 fast speed @ 1.8V pullup"
io8_ft_v33_fs_pd_1v8  "IO8_FT_V33 fast speed @ 1.8V pulldown"
io8_ft_v33_ms_1v8  "IO8_FT_V33 med speed @ 1.8V"
io8_ft_v33_ms_pu_1v8  "IO8_FT_V33 med speed @ 1.8V pullup"
io8_ft_v33_ms_pd_1v8  "IO8_FT_V33 med speed @ 1.8V pulldown"
io8_ft_v33_ls_1v8  "IO8_FT_V33 low speed @ 1.8V"
io8_ft_v33_ls_pu_1v8  "IO8_FT_V33 low speed @ 1.8V pullup"
io8_ft_v33_ls_pd_1v8  "IO8_FT_V33 low speed @ 1.8V pulldown"
io8_ft_v33_hs_3v3  "IO8_FT_V33 high speed @ 3.3V"
io8_ft_v33_hs_pu_3v3  "IO8_FT_V33 high speed @ 3.3V pullup"
io8_ft_v33_hs_pd_3v3  "IO8_FT_V33 high speed @ 3.3V pulldown"
io8_ft_v33_fs_3v3  "IO8_FT_V33 fast speed @ 3.3V"
io8_ft_v33_fs_pu_3v3  "IO8_FT_V33 fast speed @ 3.3V pullup"
io8_ft_v33_fs_pd_3v3  "IO8_FT_V33 fast speed @ 3.3V pulldown"
io8_ft_v33_ms_3v3  "IO8_FT_V33 med speed @ 3.3V"
io8_ft_v33_ms_pu_3v3  "IO8_FT_V33 med speed @ 3.3V pullup"
io8_ft_v33_ms_pd_3v3  "IO8_FT_V33 med speed @ 3.3V pulldown"
io8_ft_v33_ls_3v3  "IO8_FT_V33 low speed @ 3.3V"
io8_ft_v33_ls_pu_3v3  "IO8_FT_V33 low speed @ 3.3V pullup"
io8_ft_v33_ls_pd_3v3  "IO8_FT_V33 low speed @ 3.3V pulldown"
[Model Selector] io8_100m_usb_id
io8_100m_ft_hs_1v2  "IO8_FT 100MHz high speed @ 1.2V"
io8_100m_ft_hs_pu_1v2  "IO8_FT 100MHz high speed @ 1.2V pullup"
io8_100m_ft_hs_pd_1v2  "IO8_FT 100MHz high speed @ 1.2V pulldown"
io8_100m_ft_fs_1v2  "IO8_FT 100MHz fast speed @ 1.2V"
io8_100m_ft_fs_pu_1v2  "IO8_FT 100MHz fast speed @ 1.2V pullup"
io8_100m_ft_fs_pd_1v2  "IO8_FT 100MHz fast speed @ 1.2V pulldown"
io8_100m_ft_ms_1v2  "IO8_FT 100MHz med speed @ 1.2V"
io8_100m_ft_ms_pu_1v2  "IO8_FT 100MHz med speed @ 1.2V pullup"
io8_100m_ft_ms_pd_1v2  "IO8_FT 100MHz med speed @ 1.2V pulldown"
io8_100m_ft_ls_1v2  "IO8_FT 100MHz low speed @ 1.2V"
io8_100m_ft_ls_pu_1v2  "IO8_FT 100MHz low speed @ 1.2V pullup"
io8_100m_ft_ls_pd_1v2  "IO8_FT 100MHz low speed @ 1.2V pulldown"
io8_100m_ft_hs_1v8  "IO8_FT 100MHz high speed @ 1.8V"
io8_100m_ft_hs_pu_1v8  "IO8_FT 100MHz high speed @ 1.8V pullup"
io8_100m_ft_hs_pd_1v8  "IO8_FT 100MHz high speed @ 1.8V pulldown"
io8_100m_ft_fs_1v8  "IO8_FT 100MHz fast speed @ 1.8V"
io8_100m_ft_fs_pu_1v8  "IO8_FT 100MHz fast speed @ 1.8V pullup"
io8_100m_ft_fs_pd_1v8  "IO8_FT 100MHz fast speed @ 1.8V pulldown"
io8_100m_ft_ms_1v8  "IO8_FT 100MHz med speed @ 1.8V"
io8_100m_ft_ms_pu_1v8  "IO8_FT 100MHz med speed @ 1.8V pullup"
io8_100m_ft_ms_pd_1v8  "IO8_FT 100MHz med speed @ 1.8V pulldown"
io8_100m_ft_ls_1v8  "IO8_FT 100MHz low speed @ 1.8V"
io8_100m_ft_ls_pu_1v8  "IO8_FT 100MHz low speed @ 1.8V pullup"
io8_100m_ft_ls_pd_1v8  "IO8_FT 100MHz low speed @ 1.8V pulldown"
io8_100m_ft_hs_3v3  "IO8_FT 100MHz high speed @ 3.3V"
io8_100m_ft_hs_pu_3v3  "IO8_FT 100MHz high speed @ 3.3V pullup"
io8_100m_ft_hs_pd_3v3  "IO8_FT 100MHz high speed @ 3.3V pulldown"
io8_100m_ft_fs_3v3  "IO8_FT 100MHz fast speed @ 3.3V"
io8_100m_ft_fs_pu_3v3  "IO8_FT 100MHz fast speed @ 3.3V pullup"
io8_100m_ft_fs_pd_3v3  "IO8_FT 100MHz fast speed @ 3.3V pulldown"
io8_100m_ft_ms_3v3  "IO8_FT 100MHz med speed @ 3.3V"
io8_100m_ft_ms_pu_3v3  "IO8_FT 100MHz med speed @ 3.3V pullup"
io8_100m_ft_ms_pd_3v3  "IO8_FT 100MHz med speed @ 3.3V pulldown"
io8_100m_ft_ls_3v3  "IO8_FT 100MHz low speed @ 3.3V"
io8_100m_ft_ls_pu_3v3  "IO8_FT 100MHz low speed @ 3.3V pullup"
io8_100m_ft_ls_pd_3v3  "IO8_FT 100MHz low speed @ 3.3V pulldown"
io8usb_id_nopu  "IOUSB ID @ 3.3V"
io8usb_id_pu  "IOUSB ID @ 3.3V pullup"
[Model Selector] io8_100m_usb_vbus_ft
io8_100m_ft_hs_1v2  "IO8_FT 100MHz high speed @ 1.2V"
io8_100m_ft_hs_pu_1v2  "IO8_FT 100MHz high speed @ 1.2V pullup"
io8_100m_ft_hs_pd_1v2  "IO8_FT 100MHz high speed @ 1.2V pulldown"
io8_100m_ft_fs_1v2  "IO8_FT 100MHz fast speed @ 1.2V"
io8_100m_ft_fs_pu_1v2  "IO8_FT 100MHz fast speed @ 1.2V pullup"
io8_100m_ft_fs_pd_1v2  "IO8_FT 100MHz fast speed @ 1.2V pulldown"
io8_100m_ft_ms_1v2  "IO8_FT 100MHz med speed @ 1.2V"
io8_100m_ft_ms_pu_1v2  "IO8_FT 100MHz med speed @ 1.2V pullup"
io8_100m_ft_ms_pd_1v2  "IO8_FT 100MHz med speed @ 1.2V pulldown"
io8_100m_ft_ls_1v2  "IO8_FT 100MHz low speed @ 1.2V"
io8_100m_ft_ls_pu_1v2  "IO8_FT 100MHz low speed @ 1.2V pullup"
io8_100m_ft_ls_pd_1v2  "IO8_FT 100MHz low speed @ 1.2V pulldown"
io8_100m_ft_hs_1v8  "IO8_FT 100MHz high speed @ 1.8V"
io8_100m_ft_hs_pu_1v8  "IO8_FT 100MHz high speed @ 1.8V pullup"
io8_100m_ft_hs_pd_1v8  "IO8_FT 100MHz high speed @ 1.8V pulldown"
io8_100m_ft_fs_1v8  "IO8_FT 100MHz fast speed @ 1.8V"
io8_100m_ft_fs_pu_1v8  "IO8_FT 100MHz fast speed @ 1.8V pullup"
io8_100m_ft_fs_pd_1v8  "IO8_FT 100MHz fast speed @ 1.8V pulldown"
io8_100m_ft_ms_1v8  "IO8_FT 100MHz med speed @ 1.8V"
io8_100m_ft_ms_pu_1v8  "IO8_FT 100MHz med speed @ 1.8V pullup"
io8_100m_ft_ms_pd_1v8  "IO8_FT 100MHz med speed @ 1.8V pulldown"
io8_100m_ft_ls_1v8  "IO8_FT 100MHz low speed @ 1.8V"
io8_100m_ft_ls_pu_1v8  "IO8_FT 100MHz low speed @ 1.8V pullup"
io8_100m_ft_ls_pd_1v8  "IO8_FT 100MHz low speed @ 1.8V pulldown"
io8_100m_ft_hs_3v3  "IO8_FT 100MHz high speed @ 3.3V"
io8_100m_ft_hs_pu_3v3  "IO8_FT 100MHz high speed @ 3.3V pullup"
io8_100m_ft_hs_pd_3v3  "IO8_FT 100MHz high speed @ 3.3V pulldown"
io8_100m_ft_fs_3v3  "IO8_FT 100MHz fast speed @ 3.3V"
io8_100m_ft_fs_pu_3v3  "IO8_FT 100MHz fast speed @ 3.3V pullup"
io8_100m_ft_fs_pd_3v3  "IO8_FT 100MHz fast speed @ 3.3V pulldown"
io8_100m_ft_ms_3v3  "IO8_FT 100MHz med speed @ 3.3V"
io8_100m_ft_ms_pu_3v3  "IO8_FT 100MHz med speed @ 3.3V pullup"
io8_100m_ft_ms_pd_3v3  "IO8_FT 100MHz med speed @ 3.3V pulldown"
io8_100m_ft_ls_3v3  "IO8_FT 100MHz low speed @ 3.3V"
io8_100m_ft_ls_pu_3v3  "IO8_FT 100MHz low speed @ 3.3V pullup"
io8_100m_ft_ls_pd_3v3  "IO8_FT 100MHz low speed @ 3.3V pulldown"
io8usb_adp "IOUSB ADP @ 3.3V"
io8usb_vbus "IOUSB VBUS @ 3.3V"
[Model Selector] io8_usb_ft
io8_100m_ft_hs_1v2  "IO8_FT 100MHz high speed @ 1.2V"
io8_100m_ft_hs_pu_1v2  "IO8_FT 100MHz high speed @ 1.2V pullup"
io8_100m_ft_hs_pd_1v2  "IO8_FT 100MHz high speed @ 1.2V pulldown"
io8_100m_ft_fs_1v2  "IO8_FT 100MHz fast speed @ 1.2V"
io8_100m_ft_fs_pu_1v2  "IO8_FT 100MHz fast speed @ 1.2V pullup"
io8_100m_ft_fs_pd_1v2  "IO8_FT 100MHz fast speed @ 1.2V pulldown"
io8_100m_ft_ms_1v2  "IO8_FT 100MHz med speed @ 1.2V"
io8_100m_ft_ms_pu_1v2  "IO8_FT 100MHz med speed @ 1.2V pullup"
io8_100m_ft_ms_pd_1v2  "IO8_FT 100MHz med speed @ 1.2V pulldown"
io8_100m_ft_ls_1v2  "IO8_FT 100MHz low speed @ 1.2V"
io8_100m_ft_ls_pu_1v2  "IO8_FT 100MHz low speed @ 1.2V pullup"
io8_100m_ft_ls_pd_1v2  "IO8_FT 100MHz low speed @ 1.2V pulldown"
io8_100m_ft_hs_1v8  "IO8_FT 100MHz high speed @ 1.8V"
io8_100m_ft_hs_pu_1v8  "IO8_FT 100MHz high speed @ 1.8V pullup"
io8_100m_ft_hs_pd_1v8  "IO8_FT 100MHz high speed @ 1.8V pulldown"
io8_100m_ft_fs_1v8  "IO8_FT 100MHz fast speed @ 1.8V"
io8_100m_ft_fs_pu_1v8  "IO8_FT 100MHz fast speed @ 1.8V pullup"
io8_100m_ft_fs_pd_1v8  "IO8_FT 100MHz fast speed @ 1.8V pulldown"
io8_100m_ft_ms_1v8  "IO8_FT 100MHz med speed @ 1.8V"
io8_100m_ft_ms_pu_1v8  "IO8_FT 100MHz med speed @ 1.8V pullup"
io8_100m_ft_ms_pd_1v8  "IO8_FT 100MHz med speed @ 1.8V pulldown"
io8_100m_ft_ls_1v8  "IO8_FT 100MHz low speed @ 1.8V"
io8_100m_ft_ls_pu_1v8  "IO8_FT 100MHz low speed @ 1.8V pullup"
io8_100m_ft_ls_pd_1v8  "IO8_FT 100MHz low speed @ 1.8V pulldown"
io8_100m_ft_hs_3v3  "IO8_FT 100MHz high speed @ 3.3V"
io8_100m_ft_hs_pu_3v3  "IO8_FT 100MHz high speed @ 3.3V pullup"
io8_100m_ft_hs_pd_3v3  "IO8_FT 100MHz high speed @ 3.3V pulldown"
io8_100m_ft_fs_3v3  "IO8_FT 100MHz fast speed @ 3.3V"
io8_100m_ft_fs_pu_3v3  "IO8_FT 100MHz fast speed @ 3.3V pullup"
io8_100m_ft_fs_pd_3v3  "IO8_FT 100MHz fast speed @ 3.3V pulldown"
io8_100m_ft_ms_3v3  "IO8_FT 100MHz med speed @ 3.3V"
io8_100m_ft_ms_pu_3v3  "IO8_FT 100MHz med speed @ 3.3V pullup"
io8_100m_ft_ms_pd_3v3  "IO8_FT 100MHz med speed @ 3.3V pulldown"
io8_100m_ft_ls_3v3  "IO8_FT 100MHz low speed @ 3.3V"
io8_100m_ft_ls_pu_3v3  "IO8_FT 100MHz low speed @ 3.3V pullup"
io8_100m_ft_ls_pd_3v3  "IO8_FT 100MHz low speed @ 3.3V pulldown"
io8_usb_fs_3v3  "IOUSB fast speed @ 3.3V"
io8_usb_fs_pu1_3v3  "IO8USB fast speed @ 3.3V pullup1"
io8_usb_fs_pd1_3v3  "IOUSB fast speed @ 3.3V pulldown1"
io8_usb_ls_3v3  "IOUSB low speed @ 3.3V"
io8_usb_ls_pu1_3v3  "IOUSB low speed @ 3.3V pullup1"
io8_usb_ls_pd1_3v3  "IOUSB low speed @ 3.3V pulldown1"
io8_usb_fs_pu2_3v3  "IOUSB fast speed @ 3.3V pullup2"
io8_usb_fs_pd2_3v3  "IOUSB fast speed @ 3.3V pulldown2"
io8_usb_ls_pu2_3v3  "IOUSB low speed @ 3.3V pullup2"
io8_usb_ls_pd2_3v3  "IOUSB low speed @ 3.3V pulldown2"
[Model Selector] io8_100m_i2c_ft
io8_100m_ft_hs_1v2  "IO8_FT 100MHz high speed @ 1.2V"
io8_100m_ft_hs_pu_1v2  "IO8_FT 100MHz high speed @ 1.2V pullup"
io8_100m_ft_hs_pd_1v2  "IO8_FT 100MHz high speed @ 1.2V pulldown"
io8_100m_ft_fs_1v2  "IO8_FT 100MHz fast speed @ 1.2V"
io8_100m_ft_fs_pu_1v2  "IO8_FT 100MHz fast speed @ 1.2V pullup"
io8_100m_ft_fs_pd_1v2  "IO8_FT 100MHz fast speed @ 1.2V pulldown"
io8_100m_ft_ms_1v2  "IO8_FT 100MHz med speed @ 1.2V"
io8_100m_ft_ms_pu_1v2  "IO8_FT 100MHz med speed @ 1.2V pullup"
io8_100m_ft_ms_pd_1v2  "IO8_FT 100MHz med speed @ 1.2V pulldown"
io8_100m_ft_ls_1v2  "IO8_FT 100MHz low speed @ 1.2V"
io8_100m_ft_ls_pu_1v2  "IO8_FT 100MHz low speed @ 1.2V pullup"
io8_100m_ft_ls_pd_1v2  "IO8_FT 100MHz low speed @ 1.2V pulldown"
io8_100m_ft_hs_1v8  "IO8_FT 100MHz high speed @ 1.8V"
io8_100m_ft_hs_pu_1v8  "IO8_FT 100MHz high speed @ 1.8V pullup"
io8_100m_ft_hs_pd_1v8  "IO8_FT 100MHz high speed @ 1.8V pulldown"
io8_100m_ft_fs_1v8  "IO8_FT 100MHz fast speed @ 1.8V"
io8_100m_ft_fs_pu_1v8  "IO8_FT 100MHz fast speed @ 1.8V pullup"
io8_100m_ft_fs_pd_1v8  "IO8_FT 100MHz fast speed @ 1.8V pulldown"
io8_100m_ft_ms_1v8  "IO8_FT 100MHz med speed @ 1.8V"
io8_100m_ft_ms_pu_1v8  "IO8_FT 100MHz med speed @ 1.8V pullup"
io8_100m_ft_ms_pd_1v8  "IO8_FT 100MHz med speed @ 1.8V pulldown"
io8_100m_ft_ls_1v8  "IO8_FT 100MHz low speed @ 1.8V"
io8_100m_ft_ls_pu_1v8  "IO8_FT 100MHz low speed @ 1.8V pullup"
io8_100m_ft_ls_pd_1v8  "IO8_FT 100MHz low speed @ 1.8V pulldown"
io8_100m_ft_hs_3v3  "IO8_FT 100MHz high speed @ 3.3V"
io8_100m_ft_hs_pu_3v3  "IO8_FT 100MHz high speed @ 3.3V pullup"
io8_100m_ft_hs_pd_3v3  "IO8_FT 100MHz high speed @ 3.3V pulldown"
io8_100m_ft_fs_3v3  "IO8_FT 100MHz fast speed @ 3.3V"
io8_100m_ft_fs_pu_3v3  "IO8_FT 100MHz fast speed @ 3.3V pullup"
io8_100m_ft_fs_pd_3v3  "IO8_FT 100MHz fast speed @ 3.3V pulldown"
io8_100m_ft_ms_3v3  "IO8_FT 100MHz med speed @ 3.3V"
io8_100m_ft_ms_pu_3v3  "IO8_FT 100MHz med speed @ 3.3V pullup"
io8_100m_ft_ms_pd_3v3  "IO8_FT 100MHz med speed @ 3.3V pulldown"
io8_100m_ft_ls_3v3  "IO8_FT 100MHz low speed @ 3.3V"
io8_100m_ft_ls_pu_3v3  "IO8_FT 100MHz low speed @ 3.3V pullup"
io8_100m_ft_ls_pd_3v3  "IO8_FT 100MHz low speed @ 3.3V pulldown"
io8_100m_i2c_ft_1v2  "IO8_FT 100MHz I2C @ 1.2V"
io8_100m_i2c_ft_pu_1v2  "IO8_FT 100MHz I2C @ 1.2V pullup"
io8_100m_i2c_ft_pd_1v2  "IO8_FT 100MHz I2C @ 1.2V pulldown"
io8_100m_i2c_ft_1v8  "IO8_FT 100MHz I2C @ 1.8V"
io8_100m_i2c_ft_pu_1v8  "IO8_FT 100MHz I2C @ 1.8V pullup"
io8_100m_i2c_ft_pd_1v8  "IO8_FT 100MHz I2C @ 1,8V pulldown"
io8_100m_i2c_ft_3v3  "IO8_FT 100MHz I2C @ 3.3V"
io8_100m_i2c_ft_pu_3v3  "IO8_FT 100MHz I2C HSLV @ 3.3V pullup"
io8_100m_i2c_ft_pd_3v3  "IO8_FT 100MHz I2C @ 3.3V pulldown"
[Model Selector] io8_166m_hslv_i2c_ft
io8_166m_ft_hs_1v2  "IO8_FT 166MHz high speed @ 1.2V"
io8_166m_ft_hs_pu_1v2  "IO8_FT 166MHz high speed @ 1.2V pullup"
io8_166m_ft_hs_pd_1v2  "IO8_FT 166MHz high speed @ 1.2V pulldown"
io8_166m_ft_fs_1v2  "IO8_FT 166MHz fast speed @ 1.2V"
io8_166m_ft_fs_pu_1v2  "IO8_FT 166MHz fast speed @ 1.2V pullup"
io8_166m_ft_fs_pd_1v2  "IO8_FT 166MHz fast speed @ 1.2V pulldown"
io8_166m_ft_ms_1v2  "IO8_FT 166MHz med speed @ 1.2V"
io8_166m_ft_ms_pu_1v2  "IO8_FT 166MHz med speed @ 1.2V pullup"
io8_166m_ft_ms_pd_1v2  "IO8_FT 166MHz med speed @ 1.2V pulldown"
io8_166m_ft_ls_1v2  "IO8_FT 166MHz low speed @ 1.2V"
io8_166m_ft_ls_pu_1v2  "IO8_FT 166MHz low speed @ 1.2V pullup"
io8_166m_ft_ls_pd_1v2  "IO8_FT 166MHz low speed @ 1.2V pulldown"
io8_166m_ft_hs_1v8  "IO8_FT 166MHz high speed @ 1.8V"
io8_166m_ft_hs_pu_1v8  "IO8_FT 166MHz high speed @ 1.8V pullup"
io8_166m_ft_hs_pd_1v8  "IO8_FT 166MHz high speed @ 1.8V pulldown"
io8_166m_ft_fs_1v8  "IO8_FT 166MHz fast speed @ 1.8V"
io8_166m_ft_fs_pu_1v8  "IO8_FT 166MHz fast speed @ 1.8V pullup"
io8_166m_ft_fs_pd_1v8  "IO8_FT 166MHz fast speed @ 1.8V pulldown"
io8_166m_ft_ms_1v8  "IO8_FT 166MHz med speed @ 1.8V"
io8_166m_ft_ms_pu_1v8  "IO8_FT 166MHz med speed @ 1.8V pullup"
io8_166m_ft_ms_pd_1v8  "IO8_FT 166MHz med speed @ 1.8V pulldown"
io8_166m_ft_ls_1v8  "IO8_FT 166MHz low speed @ 1.8V"
io8_166m_ft_ls_pu_1v8  "IO8_FT 166MHz low speed @ 1.8V pullup"
io8_166m_ft_ls_pd_1v8  "IO8_FT 166MHz low speed @ 1.8V pulldown"
io8_166m_ft_hs_3v3  "IO8_FT 166MHz high speed @ 3.3V"
io8_166m_ft_hs_pu_3v3  "IO8_FT 166MHz high speed @ 3.3V pullup"
io8_166m_ft_hs_pd_3v3  "IO8_FT 166MHz high speed @ 3.3V pulldown"
io8_166m_ft_fs_3v3  "IO8_FT 166MHz fast speed @ 3.3V"
io8_166m_ft_fs_pu_3v3  "IO8_FT 166MHz fast speed @ 3.3V pullup"
io8_166m_ft_fs_pd_3v3  "IO8_FT 166MHz fast speed @ 3.3V pulldown"
io8_166m_ft_ms_3v3  "IO8_FT 166MHz med speed @ 3.3V"
io8_166m_ft_ms_pu_3v3  "IO8_FT 166MHz med speed @ 3.3V pullup"
io8_166m_ft_ms_pd_3v3  "IO8_FT 166MHz med speed @ 3.3V pulldown"
io8_166m_ft_ls_3v3  "IO8_FT 166MHz low speed @ 3.3V"
io8_166m_ft_ls_pu_3v3  "IO8_FT 166MHz low speed @ 3.3V pullup"
io8_166m_ft_ls_pd_3v3  "IO8_FT 166MHz low speed @ 3.3V pulldown"
io8_166m_hslv_ft_hs_1v2  "IO8_FT 166MHz HSLV high speed @ 1.2V"
io8_166m_hslv_ft_hs_pu_1v2  "IO8_FT 166MHz HSLV high speed @ 1.2V pullup"
io8_166m_hslv_ft_hs_pd_1v2  "IO8_FT 166MHz HSLV high speed @ 1.2V pulldown"
io8_166m_hslv_ft_fs_1v2  "IO8_FT 166MHz HSLV fast speed @ 1.2V"
io8_166m_hslv_ft_fs_pu_1v2  "IO8_FT 166MHz HSLV fast speed @ 1.2V pullup"
io8_166m_hslv_ft_fs_pd_1v2  "IO8_FT 166MHz HSLV fast speed @ 1.2V pulldown"
io8_166m_hslv_ft_ms_1v2  "IO8_FT 166MHz HSLV med speed @ 1.2V"
io8_166m_hslv_ft_ms_pu_1v2  "IO8_FT 166MHz HSLV med speed @ 1.2V pullup"
io8_166m_hslv_ft_ms_pd_1v2  "IO8_FT 166MHz HSLV med speed @ 1.2V pulldown"
io8_166m_hslv_ft_ls_1v2  "IO8_FT 166MHz HSLV low speed @ 1.2V"
io8_166m_hslv_ft_ls_pu_1v2  "IO8_FT 166MHz HSLV low speed @ 1.2V pullup"
io8_166m_hslv_ft_ls_pd_1v2  "IO8_FT 166MHz HSLV low speed @ 1.2V pulldown"
io8_166m_hslv_ft_hs_1v8  "IO8_FT 166MHz HSLV high speed @ 1.8V"
io8_166m_hslv_ft_hs_pu_1v8  "IO8_FT 166MHz HSLV high speed @ 1.8V pullup"
io8_166m_hslv_ft_hs_pd_1v8  "IO8_FT 166MHz HSLV high speed @ 1.8V pulldown"
io8_166m_hslv_ft_fs_1v8  "IO8_FT 166MHz HSLV fast speed @ 1.8V"
io8_166m_hslv_ft_fs_pu_1v8  "IO8_FT 166MHz HSLV fast speed @ 1.8V pullup"
io8_166m_hslv_ft_fs_pd_1v8  "IO8_FT 166MHz HSLV fast speed @ 1.8V pulldown"
io8_166m_hslv_ft_ms_1v8  "IO8_FT 166MHz HSLV med speed @ 1.8V"
io8_166m_hslv_ft_ms_pu_1v8  "IO8_FT 166MHz HSLV med speed @ 1.8V pullup"
io8_166m_hslv_ft_ms_pd_1v8  "IO8_FT 166MHz HSLV med speed @ 1.8V pulldown"
io8_166m_hslv_ft_ls_1v8  "IO8_FT 166MHz HSLV low speed @ 1.8V"
io8_166m_hslv_ft_ls_pu_1v8  "IO8_FT 166MHz HSLV low speed @ 1.8V pullup"
io8_166m_hslv_ft_ls_pd_1v8  "IO8_FT 166MHz HSLV low speed @ 1.8V pulldown"
io8_166m_hslv_ft_hs_2v5  "IO8_FT 166MHz HSLV high speed @ 2.5V"
io8_166m_hslv_ft_hs_pu_2v5  "IO8_FT 166MHz HSLV high speed @ 2.5V pullup"
io8_166m_hslv_ft_hs_pd_2v5  "IO8_FT 166MHz HSLV high speed @ 2.5V pulldown"
io8_166m_hslv_ft_fs_2v5  "IO8_FT 166MHz HSLV fast speed @ 2.5V"
io8_166m_hslv_ft_fs_pu_2v5  "IO8_FT 166MHz HSLV fast speed @ 2.5V pullup"
io8_166m_hslv_ft_fs_pd_2v5  "IO8_FT 166MHz HSLV fast speed @ 2.5V pulldown"
io8_166m_hslv_ft_ms_2v5  "IO8_FT 166MHz HSLV med speed @ 2.5V"
io8_166m_hslv_ft_ms_pu_2v5  "IO8_FT 166MHz HSLV med speed @ 2.5V pullup"
io8_166m_hslv_ft_ms_pd_2v5  "IO8_FT 166MHz HSLV med speed @ 2.5V pulldown"
io8_166m_hslv_ft_ls_2v5  "IO8_FT 166MHz HSLV low speed @ 2.5V"
io8_166m_hslv_ft_ls_pu_2v5  "IO8_FT 166MHz HSLV low speed @ 2.5V pullup"
io8_166m_hslv_ft_ls_pd_2v5  "IO8_FT 166MHz HSLV low speed @ 2.5V pulldown"
io8_166m_i2c_ft_1v2  "IO8_FT 166MHz I2C @ 1.2V"
io8_166m_i2c_ft_pu_1v2  "IO8_FT 166MHz I2C @ 1.2V pullup"
io8_166m_i2c_ft_pd_1v2  "IO8_FT 166MHz I2C @ 1.2V pulldown"
io8_166m_i2c_ft_1v8  "IO8_FT 166MHz I2C @ 1.8V"
io8_166m_i2c_ft_pu_1v8  "IO8_FT 166MHz I2C @ 1.8V pullup"
io8_166m_i2c_ft_pd_1v8  "IO8_FT 166MHz I2C @ 1,8V pulldown"
io8_166m_i2c_ft_3v3  "IO8_FT 166MHz I2C @ 3.3V"
io8_166m_i2c_ft_pu_3v3  "IO8_FT 166MHz I2C HSLV @ 3.3V pullup"
io8_166m_i2c_ft_pd_3v3  "IO8_FT 166MHz I2C @ 3.3V pulldown"
| Models and submodels in the file (212): io8_100m_ft_hs_1v2 (I/O), io8_100m_ft_hs_pu_1v2 (I/O), io8_100m_ft_hs_pd_1v2 (I/O), io8_100m_ft_fs_1v2 (I/O), io8_100m_ft_fs_pu_1v2 (I/O), io8_100m_ft_fs_pd_1v2 (I/O), io8_100m_ft_ms_1v2 (I/O), io8_100m_ft_ms_pu_1v2 (I/O), io8_100m_ft_ms_pd_1v2 (I/O), io8_100m_ft_ls_1v2 (I/O), io8_100m_ft_ls_pu_1v2 (I/O), io8_100m_ft_ls_pd_1v2 (I/O), io8_100m_ft_hs_1v8 (I/O), io8_100m_ft_hs_pu_1v8 (I/O), io8_100m_ft_hs_pd_1v8 (I/O), io8_100m_ft_fs_1v8 (I/O), io8_100m_ft_fs_pu_1v8 (I/O), io8_100m_ft_fs_pd_1v8 (I/O), io8_100m_ft_ms_1v8 (I/O), io8_100m_ft_ms_pu_1v8 (I/O), io8_100m_ft_ms_pd_1v8 (I/O), io8_100m_ft_ls_1v8 (I/O), io8_100m_ft_ls_pu_1v8 (I/O), io8_100m_ft_ls_pd_1v8 (I/O), io8_100m_ft_hs_3v3 (I/O), io8_100m_ft_hs_pu_3v3 (I/O), io8_100m_ft_hs_pd_3v3 (I/O), io8_100m_ft_fs_3v3 (I/O), io8_100m_ft_fs_pu_3v3 (I/O), io8_100m_ft_fs_pd_3v3 (I/O), io8_100m_ft_ms_3v3 (I/O), io8_100m_ft_ms_pu_3v3 (I/O), io8_100m_ft_ms_pd_3v3 (I/O), io8_100m_ft_ls_3v3 (I/O), io8_100m_ft_ls_pu_3v3 (I/O), io8_100m_ft_ls_pd_3v3 (I/O), io8_100m_hslv_ft_hs_1v2 (I/O), io8_100m_hslv_ft_hs_pu_1v2 (I/O), io8_100m_hslv_ft_hs_pd_1v2 (I/O), io8_100m_hslv_ft_fs_1v2 (I/O), io8_100m_hslv_ft_fs_pu_1v2 (I/O), io8_100m_hslv_ft_fs_pd_1v2 (I/O), io8_100m_hslv_ft_ms_1v2 (I/O), io8_100m_hslv_ft_ms_pu_1v2 (I/O), io8_100m_hslv_ft_ms_pd_1v2 (I/O), io8_100m_hslv_ft_ls_1v2 (I/O), io8_100m_hslv_ft_ls_pu_1v2 (I/O), io8_100m_hslv_ft_ls_pd_1v2 (I/O), io8_100m_hslv_ft_hs_1v8 (I/O), io8_100m_hslv_ft_hs_pu_1v8 (I/O), io8_100m_hslv_ft_hs_pd_1v8 (I/O), io8_100m_hslv_ft_fs_1v8 (I/O), io8_100m_hslv_ft_fs_pu_1v8 (I/O), io8_100m_hslv_ft_fs_pd_1v8 (I/O), io8_100m_hslv_ft_ms_1v8 (I/O), io8_100m_hslv_ft_ms_pu_1v8 (I/O), io8_100m_hslv_ft_ms_pd_1v8 (I/O), io8_100m_hslv_ft_ls_1v8 (I/O), io8_100m_hslv_ft_ls_pu_1v8 (I/O), io8_100m_hslv_ft_ls_pd_1v8 (I/O), io8_100m_hslv_ft_hs_2v5 (I/O), io8_100m_hslv_ft_hs_pu_2v5 (I/O), io8_100m_hslv_ft_hs_pd_2v5 (I/O), io8_100m_hslv_ft_fs_2v5 (I/O), io8_100m_hslv_ft_fs_pu_2v5 (I/O), io8_100m_hslv_ft_fs_pd_2v5 (I/O), io8_100m_hslv_ft_ms_2v5 (I/O), io8_100m_hslv_ft_ms_pu_2v5 (I/O), io8_100m_hslv_ft_ms_pd_2v5 (I/O), io8_100m_hslv_ft_ls_2v5 (I/O), io8_100m_hslv_ft_ls_pu_2v5 (I/O), io8_100m_hslv_ft_ls_pd_2v5 (I/O), io8_166m_ft_hs_1v2 (I/O), io8_166m_ft_hs_pu_1v2 (I/O), io8_166m_ft_hs_pd_1v2 (I/O), io8_166m_ft_fs_1v2 (I/O), io8_166m_ft_fs_pu_1v2 (I/O), io8_166m_ft_fs_pd_1v2 (I/O), io8_166m_ft_ms_1v2 (I/O), io8_166m_ft_ms_pu_1v2 (I/O)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
